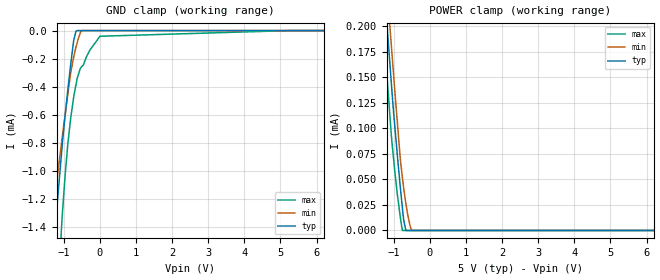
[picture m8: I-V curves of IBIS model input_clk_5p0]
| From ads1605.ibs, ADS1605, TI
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|   INPUT_CLK 5.0V Model
[Model]   input_clk_5p0
Model_type   Input
Vinl = 1.5
Vinh = 3.5
|   typ   min   max
|   (nom PVT)   (Fast PVT)   (Slow PVT)
C_comp   1.179e-12   1.159e-12   1.201e-12
|Where nom PVT is NOM Process, 5.0V,39C
|   Fast PVT is Strong Process, 5.25V, -40C
|   Slow PVT is Weak Process, 4.75V, 99C
[Model Spec]
Vinl   1.5   1.425   1.575
Vinh   3.5   3.325   3.675
[Voltage Range]   5   4.75   5.25
|Ambient Temperature   25   85   -40
|Junction Temperature
[Temperature Range]   39   99   -40
[Power Clamp Reference]   5   4.75   5.25
[GND Clamp Reference]   0   0   0
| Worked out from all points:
|   GND clamp passes 1 mA (typ) near -1.10 V on its own axis
|   POWER clamp passes 1 mA (typ) near -2.76 V on its own axis
[GND Clamp]
|   Voltage   I(typ)   I(min)   I(max)
-5V       -13.46mA   -9.499mA   -24.88mA
-1.36V    -1.78mA    -1.433mA   -3.035mA
-1.246V   -1.436mA   -1.188mA   -2.401mA
-1.068V   -895.6uA   -814.7uA   -1.433mA
-962.7mV  -609uA     -604.5uA   -1.036mA
-884mV    -417.7uA   -448.5uA   -802.2uA
-820mV    -269.8uA   -321.7uA   -652.5uA
-725mV    -72.35uA   -190.3uA   -477.2uA
-626.8mV  0A         -85.69uA   -340.6uA
-520.8mV  0A         -2.654uA   -264.3uA
3.25mV    0A         0A         -40.52uA
10V       0A         0A         0A
[POWER Clamp]
|   Voltage   I(typ)   I(min)   I(max)
-5V       2.166mA    2.195mA    2.125mA
-1.33V    271.5uA    308.3uA    221.1uA
-1.21V    213uA      250uA      162.4uA
-1.173V   195.1uA    231.9uA    144.2uA
-1.1V     160.5uA    196.7uA    109.4uA
-973.2mV  103.1uA    138.5uA    58.72uA
-820mV    43.07uA    70.66uA    13.52uA
-760mV    21.78uA    51.69uA    0A
-725mV    10.36uA    41.51uA    0A
-665mV    63.03nA    26.77uA    0A
-501.8mV  0A         0A         0A
10V       0A         0A         0A
